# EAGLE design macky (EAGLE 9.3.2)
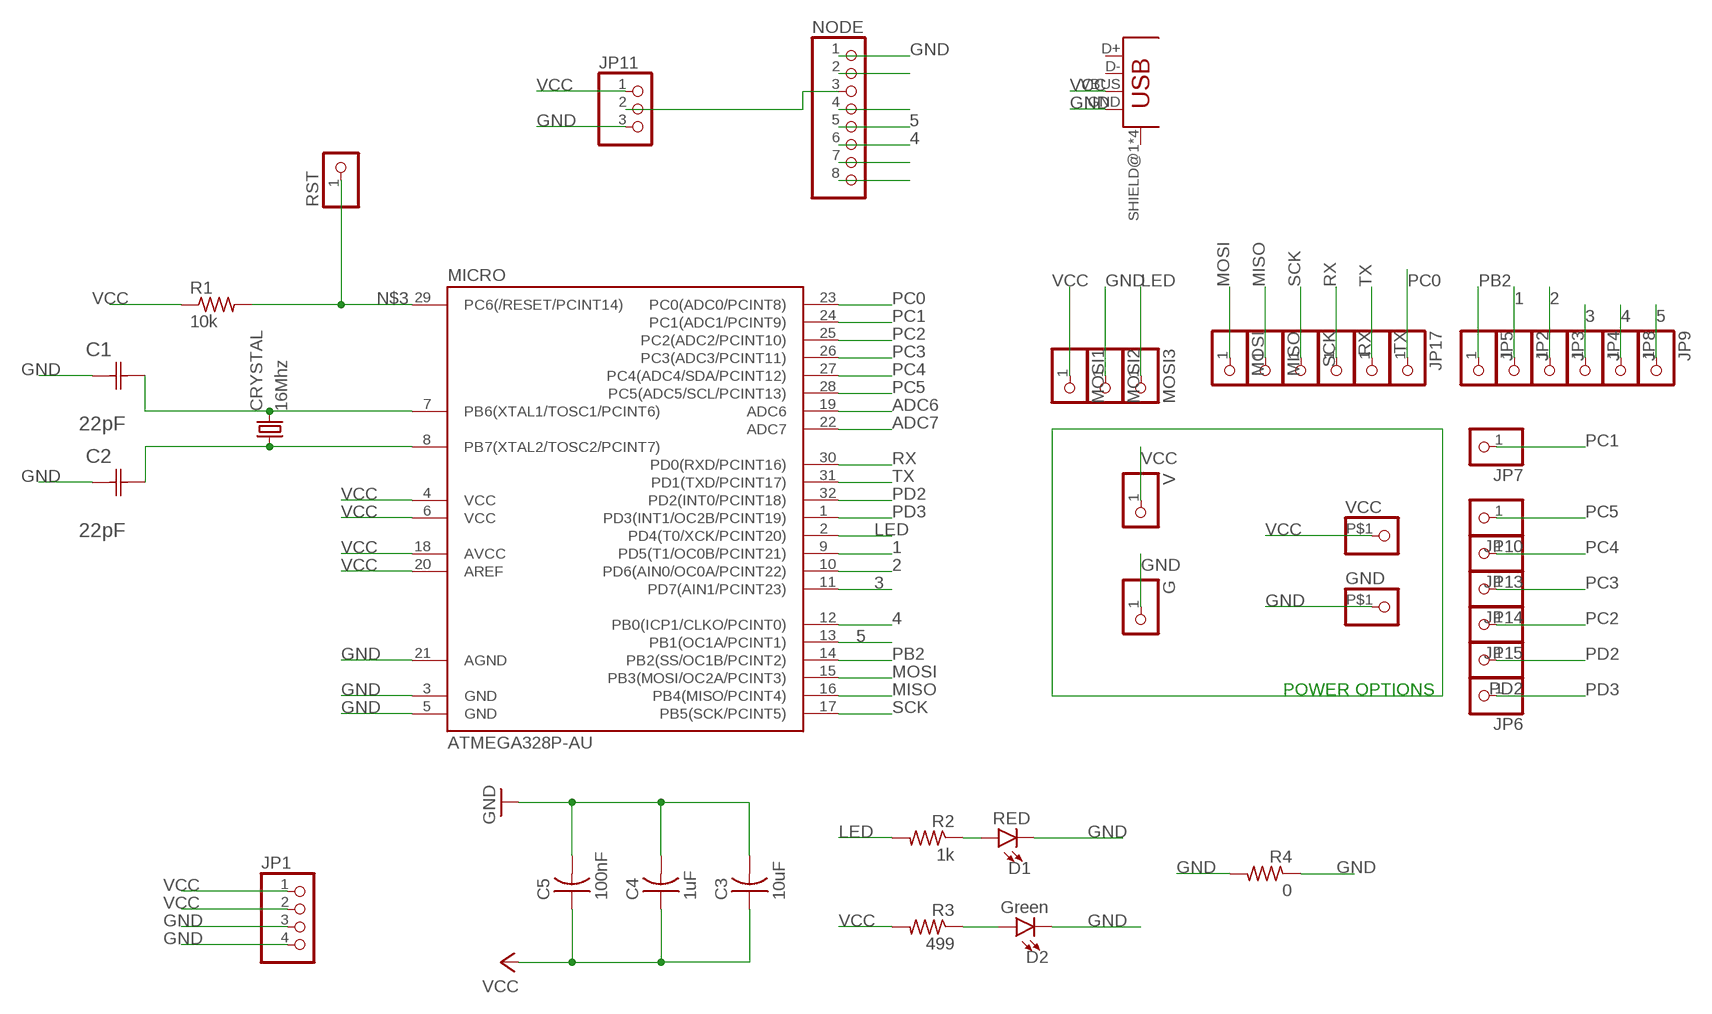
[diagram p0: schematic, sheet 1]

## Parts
C1  22pF  0612ZC225MAT2A  [CAPC3216X178N]
C2  22pF  0612ZC225MAT2A  [CAPC3216X178N]
C3  10uF  CAP-US1206FAB  [C1206FAB]
C4  1uF  CAP-US1206FAB  [C1206FAB]
C5  100nF  CAP-US1206FAB  [C1206FAB]
CRYSTAL  16Mhz  CSM-7X-DU  [CSM-7X-DU]
D1  RED  LED-RED1206  [LED-1206]
D2  Green  LED-RED1206  [LED-1206]
G  PINHD-1X1  [1X01]
GND  PINHD-1X1-BIGPOGO  [1X1-BIGPOGO]
JP1  PINHD-1X4  [1X04]
JP2  PINHD-1X1  [1X01]
JP3  PINHD-1X1  [1X01]
JP4  PINHD-1X1  [1X01]
JP5  PINHD-1X1  [1X01]
JP6  PINHD-1X1  [1X01]
JP7  PINHD-1X1  [1X01]
JP8  PINHD-1X1  [1X01]
JP9  PINHD-1X1  [1X01]
JP10  PINHD-1X1  [1X01]
JP11  PINHD-1X3  [1X03]
JP13  PINHD-1X1  [1X01]
JP14  PINHD-1X1  [1X01]
JP15  PINHD-1X1  [1X01]
JP17  PINHD-1X1  [1X01]
MICRO  ATMEGA328P-AU  ATMEGA48/88/168-AU  [TQFP32-08]
MISO  PINHD-1X1  [1X01]
MOSI  PINHD-1X1  [1X01]
MOSI1  PINHD-1X1  [1X01]
MOSI2  PINHD-1X1  [1X01]
MOSI3  PINHD-1X1  [1X01]
NODE  PINHD-1X8  [1X08]
PD2  PINHD-1X1  [1X01]
R1  10k  RES-US1206FAB  [R1206FAB]
R2  1k  RES-US1206FAB  [R1206FAB]
R3  499  RES-US1206FAB  [R1206FAB]
R4  0  RES-US1206FAB  [R1206FAB]
RST  PINHD-1X1  [1X01]
RX  PINHD-1X1  [1X01]
SCK  PINHD-1X1  [1X01]
TX  PINHD-1X1  [1X01]
U$1  USB_MINIB  [USB_MINIB]
V  PINHD-1X1  [1X01]
VCC  PINHD-1X1-BIGPOGO  [1X1-BIGPOGO]

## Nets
1: JP2.1 MICRO.9(PD5(T1/OC0B/PCINT21))
2: JP3.1 MICRO.10(PD6(AIN0/OC0A/PCINT22))
3: JP4.1 MICRO.11(PD7(AIN1/PCINT23))
4: JP8.1 MICRO.12(PB0(ICP1/CLKO/PCINT0)) NODE.6
5: JP9.1 MICRO.13(PB1(OC1A/PCINT1)) NODE.5
ADC6: MICRO.19(ADC6)
ADC7: MICRO.22(ADC7)
GND: C1.1(C1) C2.1(C1) C3.2 C4.2 C5.2 D1.C D2.C G.1 GND.P$1 JP1.3 JP1.4 JP11.3 MICRO.3(GND) MICRO.5(GND) MICRO.21(AGND) MOSI2.1 NODE.1 R4.1 R4.2 U$1.GND
LED: MICRO.2(PD4(T0/XCK/PCINT20)) MOSI3.1 R2.2
MISO: MICRO.16(PB4(MISO/PCINT4)) MISO.1
MOSI: MICRO.15(PB3(MOSI/OC2A/PCINT3)) MOSI.1
N$1: D2.A R3.1
N$2: C1.2(C2) CRYSTAL.2 MICRO.7(PB6(XTAL1/TOSC1/PCINT6))
N$3: MICRO.29(PC6(/RESET/PCINT14)) R1.2 RST.1
N$5: NODE.2
N$7: NODE.4
N$8: JP11.2 NODE.3
N$9: C2.2(C2) CRYSTAL.1 MICRO.8(PB7(XTAL2/TOSC2/PCINT7))
N$11: NODE.7
N$12: NODE.8
N$25: D1.A R2.1
PB2: JP5.1 MICRO.14(PB2(SS/OC1B/PCINT2))
PC0: JP17.1 MICRO.23(PC0(ADC0/PCINT8))
PC1: JP7.1 MICRO.24(PC1(ADC1/PCINT9))
PC2: JP15.1 MICRO.25(PC2(ADC2/PCINT10))
PC3: JP14.1 MICRO.26(PC3(ADC3/PCINT11))
PC4: JP13.1 MICRO.27(PC4(ADC4/SDA/PCINT12))
PC5: JP10.1 MICRO.28(PC5(ADC5/SCL/PCINT13))
PD2: MICRO.32(PD2(INT0/PCINT18)) PD2.1
PD3: JP6.1 MICRO.1(PD3(INT1/OC2B/PCINT19))
RX: MICRO.30(PD0(RXD/PCINT16)) RX.1
SCK: MICRO.17(PB5(SCK/PCINT5)) SCK.1
TX: MICRO.31(PD1(TXD/PCINT17)) TX.1
VCC: C3.1 C4.1 C5.1 JP1.1 JP1.2 JP11.1 MICRO.4(VCC) MICRO.6(VCC) MICRO.18(AVCC) MICRO.20(AREF) MOSI1.1 R1.1 R3.2 U$1.VBUS V.1 VCC.P$1
Unconnected: U$1.D+ U$1.D- U$1.SHIELD@1(SHIELD) U$1.SHIELD@2(SHIELD) U$1.SHIELD@3(SHIELD) U$1.SHIELD@4(SHIELD)

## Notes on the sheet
- POWER OPTIONS

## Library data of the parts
C1 C2 = AVX_By_element14_Batch_1:0612ZC225MAT2A: Capacitor 1206; MPN: 0612ZC225MAT2A; OC_FARNELL: -; OC_NEWARK: 12N3209; SUPPLIER: AVX; TOLERANCE: ±20%; VALUE: 2.2µF; VOLTAGERATING: 10V
C3-C5 = fab:CAP-US
CRYSTAL = 01_FAB_Hello:CSM-7X-DU: SMD CRYSTAL; OC_FARNELL: unknown; OC_NEWARK: unknown
D1 = SparkFun-LED:LED-RED: Red SMD LED; PROD_ID: DIO-09912
D2 = SparkFun-LED:LED-RED: Red SMD LED; PROD_ID: DIO-09912; VALUE: RED
G GND JP2-JP10 JP13-JP15 JP17 MISO MOSI MOSI1-MOSI3 PD2 RST RX SCK TX V VCC = adafruit:PINHD-1X1: Pin header 1x1 for 0.1" spacing
JP1 = pinhead:PINHD-1X4: PIN HEADER
JP11 = pinhead:PINHD-1X3: PIN HEADER
MICRO = atmega8:ATMEGA48/88/168
NODE = pinhead:PINHD-1X8: PIN HEADER
R1-R4 = fab:RES-US: Resistor (US Symbol)
U$1 = fab:USB_MINIB

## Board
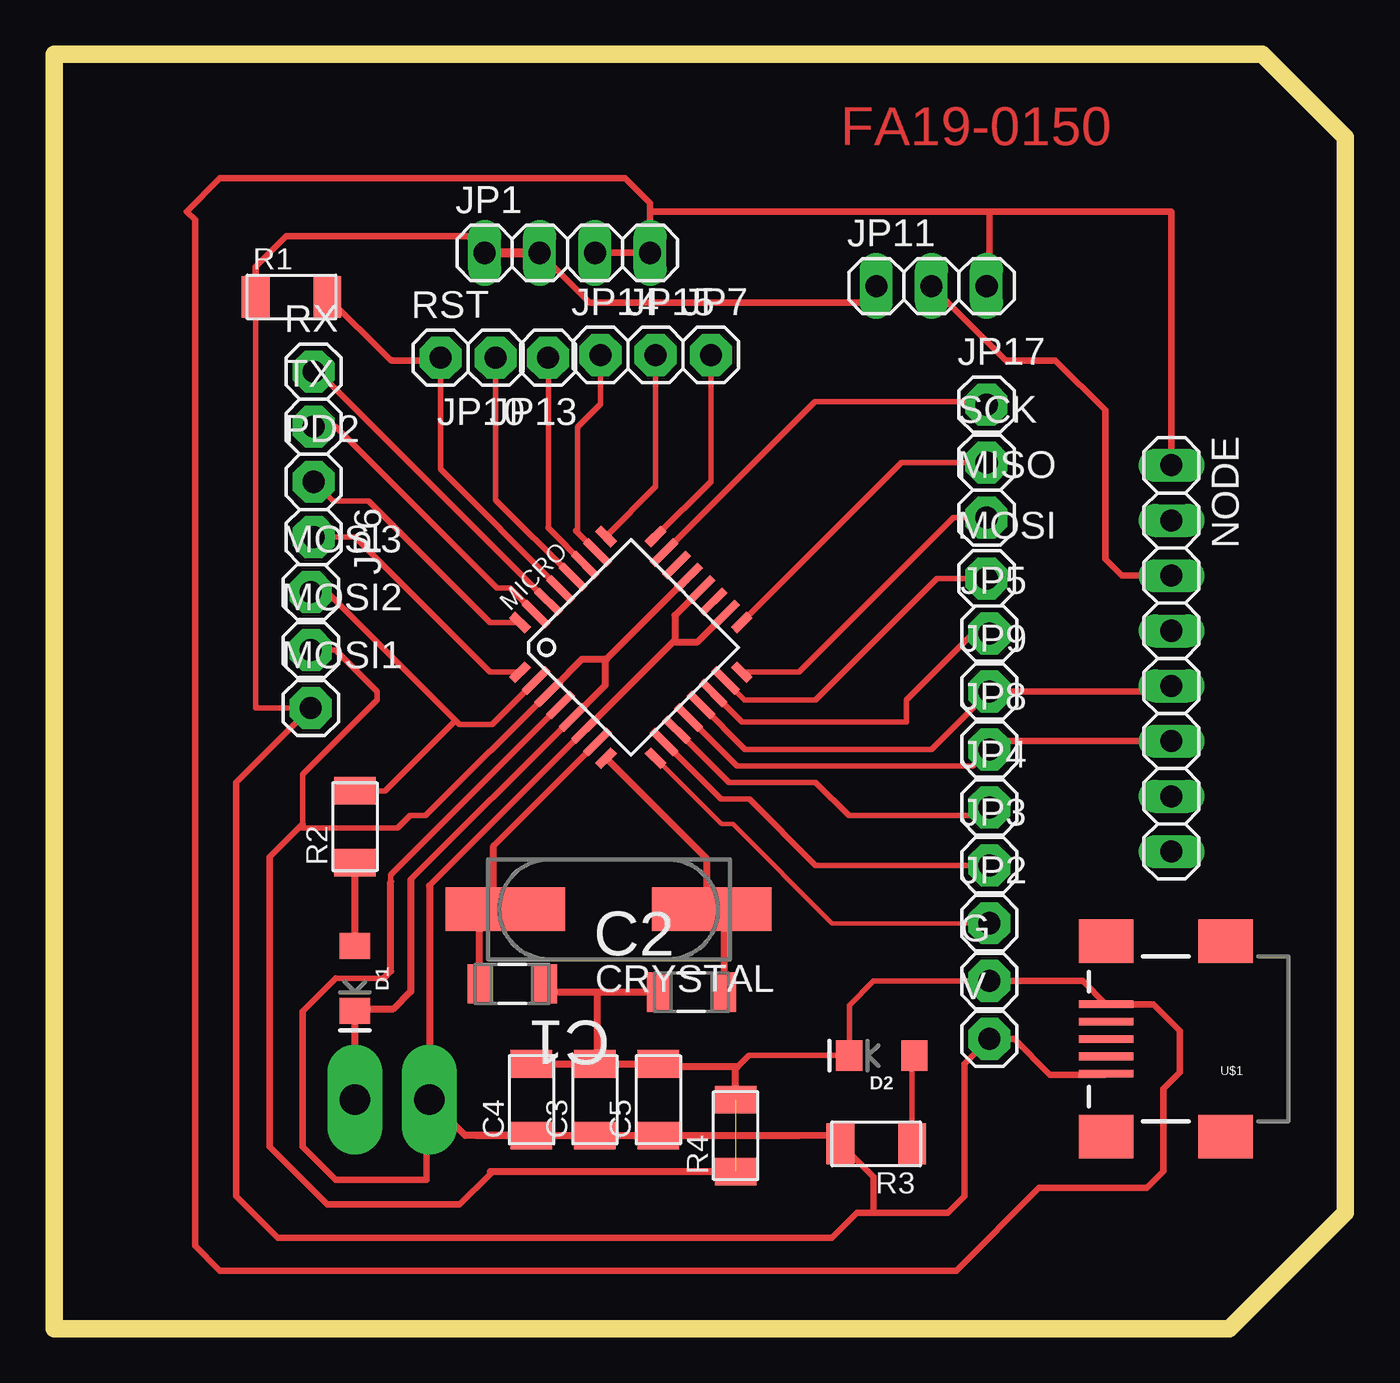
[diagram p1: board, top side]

Size 59.44 x 58.67 mm. Coordinates in mm from the lower left corner, seen from the top.
Outline: 0,58.67 0,0 54.1,0 59.44,5.33 59.44,54.86 55.63,58.67 0,58.67
Copper layers (1*16): Top 0.035mm / dielectric 1.5mm / Bottom 0.035mm
Design rules "fab (1)": minimum track width 0.3mm, minimum drill 32mil, track to track 0.315mm, track to pad 0.315mm, pad to pad 0.315mm, via to via 0.315mm, smd to smd 0.315mm, copper to edge 40mil, drill to drill 16mil, minimum pad ring 10mil, minimum via ring 8mil, stop-mask expansion 4mil, vias tented up to drill 0mil, thermal gap 10mil

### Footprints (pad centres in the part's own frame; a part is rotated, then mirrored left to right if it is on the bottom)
CAPC3216X178N = smd 1.118 x 1.803: 1 -1.499,0; 2 1.499,0
C1206FAB = smd 1.27 x 1.905: 1 -1.651,0; 2 1.651,0
CSM-7X-DU = smd 5.5 x 2: 1 -4.75,0; 2 4.75,0
LED-1206 = smd 1.2 x 1.4: A -1.5,0; C 1.5,0
1X01 = drill 1.016 pad 1.93 octagon: 1 0,0
1X1-BIGPOGO = drill 1.4 pad 2.54 long: P$1 0,0
1X04 = drill 1.016 long: 1 -3.81,0; 2 -1.27,0; 3 1.27,0; 4 3.81,0
1X03 = drill 1.016 long: 1 -2.54,0; 2 0,0; 3 2.54,0
TQFP32-08 = smd 1.016 x 0.406: 1 -4.42,2.8; 8 -4.42,-2.8; 17 4.42,-2.8; 24 4.42,2.8 | smd 1.524 x 0.356: 2 -4.166,2; 3 -4.166,1.2; 4 -4.166,0.4; 5 -4.166,-0.4; 6 -4.166,-1.2; 7 -4.166,-2; 18 4.166,-2; 19 4.166,-1.2; 20 4.166,-0.4; 21 4.166,0.4; 22 4.166,1.2; 23 4.166,2 | smd 0.406 x 1.016: 9 -2.8,-4.42; 16 2.8,-4.42; 25 2.8,4.42; 32 -2.8,4.42 | smd 0.356 x 1.524: 10 -2,-4.166; 11 -1.2,-4.166; 12 -0.4,-4.166; 13 0.4,-4.166; 14 1.2,-4.166; 15 2,-4.166; 26 2,4.166; 27 1.2,4.166; 28 0.4,4.166; 29 -0.4,4.166; 30 -1.2,4.166; 31 -2,4.166
1X08 = drill 1.016 long: 1 -8.89,0; 2 -6.35,0; 3 -3.81,0; 4 -1.27,0; 5 1.27,0; 6 3.81,0; 7 6.35,0; 8 8.89,0
R1206FAB = smd 1.27 x 1.905: 1 -1.651,0; 2 1.651,0
USB_MINIB = smd 2.5 x 0.35: D+ 3.77,0; D- 3.77,0.8; GND 3.77,-1.6; ID 3.77,-0.8; VBUS 3.77,1.6 | smd 2.5 x 2: SHIELD@1 -1.73,-4.5; SHIELD@2 -1.73,4.5; SHIELD@3 3.77,4.5; SHIELD@4 3.77,-4.5

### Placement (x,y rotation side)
C1  21.08,15.88 180 top
C2  29.34,15.49 0 top
C3  24.89,10.54 90 top
C4  21.97,10.54 90 top
C5  27.81,10.54 90 top
CRYSTAL  25.53,19.3 180 top
D1  13.84,16.13 270 top
D2  38.1,12.57 180 top
G  43.05,16 0 top
GND  13.84,10.54 90 top
JP1  23.62,49.53 0 top
JP2  43.05,18.67 0 top
JP3  43.05,21.34 0 top
JP4  43.05,24 0 top
JP5  43.05,32 0 top
JP6  11.94,36.45 269.6 top
JP7  30.23,44.83 0 top
JP8  43.05,26.67 0 top
JP9  43.05,29.34 0 top
JP10  20.32,44.7 180 top
JP11  40.39,48.01 0 top
JP13  22.73,44.7 180 top
JP14  25.15,44.83 0 top
JP15  27.69,44.83 0 top
JP17  42.93,42.55 0 top
MICRO  26.54,31.37 45 top
MISO  42.93,37.34 0 top
MOSI  42.93,34.54 0 top
MOSI1  11.81,28.58 0 top
MOSI2  11.81,31.24 0 top
MOSI3  11.81,33.91 0 top
NODE  51.44,30.86 270 top
PD2  11.94,38.99 0 top
R1  10.92,47.5 0 top
R2  13.84,23.11 90 top
R3  37.85,8.51 180 top
R4  31.37,8.89 90 top
RST  17.78,44.7 0 top
RX  11.94,44.07 0 top
SCK  42.93,39.88 0 top
TX  11.94,41.53 0 top
U$1  52.2,13.34 180 top
V  43.05,13.34 0 top
VCC  17.27,10.54 90 top

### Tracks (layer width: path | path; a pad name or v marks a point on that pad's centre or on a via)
1
  Top 0.203: MICRO.9 30.71,23.24 31.24,23.24 35.81,18.67 JP2.1
2
  Top 0.254: MICRO.10 30.7,24.38 32,24.38 35.05,21.34 JP3.1 43.81,21.34
3
  Top 0.254: JP4.1 42.86,23.81 42.67,23.62 36.58,23.62 35.05,25.15 31.07,25.15 MICRO.11
4
  Top 0.254: 42.67,25.91 42.67,26.29 JP8.1 42.29,25.91 31.44,25.91 MICRO.12
  Top 0.3: NODE.6 43.43,27.05 JP8.1
5
  Top 0.254: JP9.1 40.39,26.67 31.81,26.67 MICRO.13
  Top 0.3: JP9.1 51.18,29.34 NODE.5
GND  (1 unrouted)
  Top 0.254: G.1 37.72,16 36.6,14.88 D2.C 31.98,12.57 31.37,11.96 | 11.43,23.24 11.43,25.53 14.86,28.96 14.86,29.34 12.95,31.24 MOSI2.1 | 11.24,23.05 15.81,23.05 16.38,23.62 17.1,23.62 23.03,29.55 | MICRO.5 16.41,20.67
  Top 0.3: JP1.4 27.43,51.82 26.29,52.96 7.62,52.96 6.1,51.44 6.48,51.05 6.48,3.81 7.62,2.67 41.53,2.67 45.34,6.48 50.29,6.48 51.05,7.24 51.05,11.05 51.82,11.81 51.82,13.72 50.6,14.94 U$1.GND 47.36,16 G.1 | JP1.4 JP1.3 | NODE.1 51.44,51.44 43.05,51.44 | 43.05,51.44 27.43,51.44 JP1.4 | 43.05,51.44 43.05,48.01 | 43.43,47.62 43.05,48.01 | 43.05,48.01 JP11.3
  Top 0.305: 11.43,23.24 11.24,23.05 9.91,21.72 9.91,8.38 12.57,5.71 18.67,5.71 20.07,7.11 20.07,7.24
  Top 0.33: 13.61,14.63 D1.C | D1.C 13.46,14.25 | MICRO.3 23.03,29.55 24.3,30.82 25.36,30.82 | C1.1 22.96,15.49 25.02,15.49 | 25.02,15.49 C2.1 | GND.P$1 D1.C | D1.C 13.95,14.73 15.62,14.73 16.41,15.52 16.41,20.67 | 20.07,7.24 R4.1 | C3.2 24.76,12.32 | C4.2 C3.2 | C3.2 C5.2 27.43,12.06 31.47,12.06 31.37,11.96 R4.2 | C3.2 25.02,12.32 25.02,15.49 | 25.36,30.82 25.36,29.62 MICRO.5 | MICRO.21 25.43,30.82 25.36,30.82
LED
  Top 0.254: MOSI3.1 12.57,33.91 18.48,28 | 18.48,28 18.67,27.81 20.16,27.81 MICRO.2 | R2.2 15.24,24.77 18.48,28
MISO
  Top 0.254: MISO.1 41.4,37.34 34.29,30.22 MICRO.16
MOSI
  Top 0.254: MOSI.1 40.64,34.54 35.05,28.96 31.78,28.96 MICRO.15
N$1
  Top 0.254: R3.1 39.5,12.47 D2.A
N$2
  Top 0.254: 20.23,22.23 MICRO.7
  Top 0.33: CRYSTAL.2 20.23,18.87 | 20.23,18.87 19.56,18.34 19.56,15.37 19.58,15.39 C1.2 | 20.23,18.87 20.23,22.23
N$3
  Top 0.254: MICRO.29 17.78,39.57 RST.1
  Top 0.305: RST.1 17.78,44.58 15.6,44.58 arc-45 15.42,44.65 R1.2
N$8
  Top 0.3: JP11.2 43.81,44.58 46.1,44.58 48.39,42.29 48.39,35.43 49.15,34.67 NODE.3
N$9
  Top 0.33: MICRO.8 30.02,21.64 30.02,19.56 CRYSTAL.1 30.84,18.49 C2.2
N$25
  Top 0.33: D1.A R2.1
PB2
  Top 0.254: JP5.1 42.29,32 39.24,28.96 39.24,27.94 31.67,27.94 MICRO.14
PC0
  Top 0.254: 28.11,35.73 MICRO.23 35.02,42.67 42.8,42.67 JP17.1
PC1
  Top 0.254: JP7.1 30.23,39.01 MICRO.24
PC2
  Top 0.254: JP15.1 27.69,38.76 MICRO.25
PC3
  Top 0.254: MICRO.26 24.08,36.66 | 24.08,36.66 24,36.74 | 24.08,36.66 24.08,41.5 25.15,42.57 JP14.1
PC4
  Top 0.254: MICRO.27 22.76,36.85 | 22.76,36.85 22.73,36.88 | 22.76,36.85 22.76,44.68 JP13.1
PC5
  Top 0.254: MICRO.28 20.32,38.16 JP10.1
PD2
  Top 0.254: PD2.1 12.83,38.1 14.48,38.1 20.06,32.51 MICRO.32
PD3
  Top 0.254: JP6.1 13.84,36.45 20.07,30.22 MICRO.1
RX
  Top 0.254: MICRO.30 12.19,44.02 12.19,44.07
  Top 0.305: RX.1 12.19,44.07 12.32,44.07
SCK
  Top 0.254: MICRO.17 39.01,39.88 SCK.1
TX
  Top 0.254: TX.1 12.95,41.53 20.38,34.1 20.98,34.1 MICRO.31
VCC
  Top 0.254: R1.1 9.27,28.58 MOSI1.1 | 15.15,16.13 12.95,16.13 | MICRO.6 17.27,20.4 | 15.49,20.57 15.49,20.89 MICRO.4
  Top 0.3: JP1.2 24.64,47.24 37.08,47.24 JP11.1 | V.1 44.2,13.34 45.85,11.68 48.38,11.68 U$1.VBUS
  Top 0.305: R1.1 9.27,48.89 10.67,50.29 19.05,50.29 JP1.1 | 12.95,16.13 11.43,14.6 11.43,8.38 12.95,6.86 17.14,6.86 17.14,10.92 17.27,11.05 | MOSI1.1 8.38,25.15 8.38,6.1 10.29,4.19 35.81,4.19 36.96,5.33 37.72,5.33 | 34.29,8.89 35.81,8.89 R3.2 37.72,6.98 37.72,5.33 | 37.72,5.33 41.15,5.33 41.91,6.1 41.91,12.19 V.1
  Top 0.33: C4.1 C3.1 C5.1 34.29,8.89 | 19.43,8.89 C4.1 | 15.15,16.13 15.49,16.47 15.49,20.57 | C4.1 18.92,8.89 VCC.P$1 | MICRO.20 28.57,32.84 28.57,31.7 | 28.57,31.7 28.57,31.62 29.63,31.62 MICRO.18 | MICRO.6 28.57,31.7 | 17.27,20.4 17.27,11.05 VCC.P$1 | VCC.P$1 17.14,10.41
  Top 0.406: JP1.1 JP1.2

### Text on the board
Top: FA19-0150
